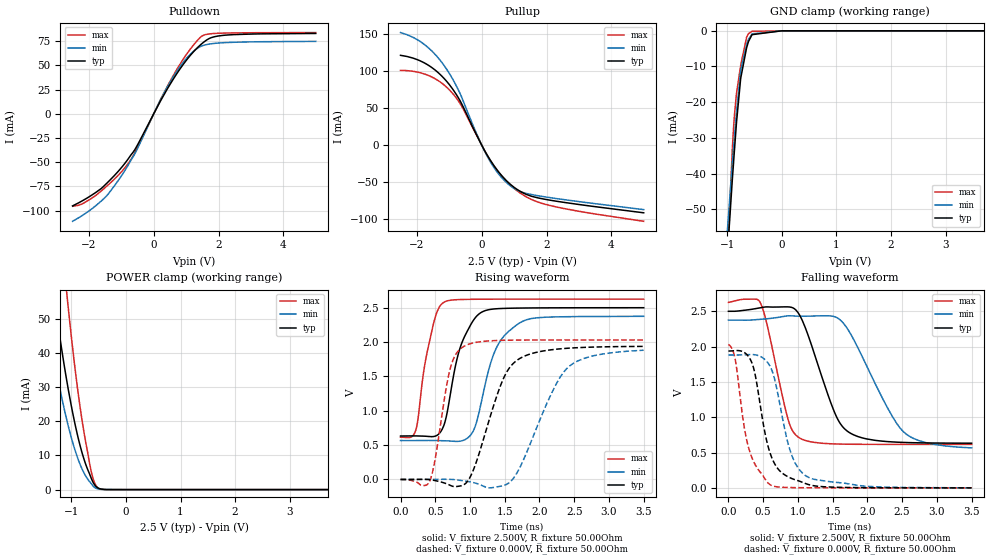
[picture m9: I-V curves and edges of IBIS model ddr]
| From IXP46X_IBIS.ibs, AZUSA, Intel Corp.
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| Note : Termination resitors may be required on pins that are lightly loaded.
|  Correlated with SPICE simulations with Standard JEDEC Test Load
|   |Vref= vcc/2 = 1.250v
|   >
|   < Rref=50ohm
|   >
|   |- Vout
|   _  Cref=30p
[Model]   ddr
Model_type   I/O
Vinl = 940.000mV
Vinh = 1.560V
Vmeas = 1.250V
Rref = 50ohm
Cref = 30.000pF
Vref = 1.250V
|   typ   min   max
C_comp   3.000pF   2.700pF   3.300pF
[Voltage Range]   2.500V   2.375V   2.625V
[Temperature Range]   25.0   110.0   -40.0
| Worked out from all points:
|   slope of the pulldown table from 0 to 0.375 V, typ, clamps not added: 16.3 ohm
|   slope of the pullup table from 0 to 0.375 V, typ, clamps not added: 13.5 ohm
|   POWER clamp passes 1 mA (typ) near -0.55 V on its own axis
|   falling waveform, V_fixture 2.500V, R_fixture 50.00Ohm: 20-80 % time 397ps typ, 564ps min, 269ps max; typ from 2.5 V to 0.632 V
|   rising waveform, V_fixture 2.500V, R_fixture 50.00Ohm: 20-80 % time 268ps typ, 316ps min, 196ps max; typ from 0.632 V to 2.5 V
|   rising waveform, V_fixture 0.000V, R_fixture 50.00Ohm: 20-80 % time 387ps typ, 500ps min, 202ps max; typ from 0 V to 1.94 V
|   falling waveform, V_fixture 0.000V, R_fixture 50.00Ohm: 20-80 % time 247ps typ, 275ps min, 219ps max; typ from 1.94 V to 0 V
[Pulldown]
|   Voltage   I(typ)   I(min)   I(max)
-2.5V     -95.15mA   -111.1mA   -95.57mA
-2.14V    -88.73mA   -103.7mA   -91.89mA
-1.46V    -72.2mA    -85.14mA   -75.16mA
-830mV    -48.59mA   -55.41mA   -53.28mA
-540mV    -34.65mA   -38.67mA   -37.31mA
205mV     12.95mA    14.13mA    14.22mA
475mV     28.81mA    30.99mA    31.72mA
915mV     51.24mA    53.39mA    56.66mA
1.3V      66.68mA    66.53mA    73.99mA
1.525V    73.57mA    70.58mA    80.96mA
1.985V    80.35mA    73.07mA    83.16mA
4.995V    82.99mA    74.82mA    83.91mA
[GND Clamp]
|   Voltage   I(typ)   I(min)   I(max)
-2.5V     -1.132A    -1.076A    -1.37A
-1.035V   -71.78mA   -63.99mA   -77.28mA
-905mV    -41.45mA   -36.81mA   -32.9mA
-885mV    -37.27mA   -33.03mA   -27.5mA
-870mV    -34.01mA   -30.32mA   -24.15mA
-830mV    -25.76mA   -22.9mA    -17.6mA
-750mV    -13.1mA    -10.79mA   -9.436mA
-645mV    -4.789mA   -3.899mA   -1.859mA
-610mV    -3.011mA   -2.375mA   -790.8uA
-545mV    -1.076mA   -850.7uA   -144.4uA
0V        -44.76nA   -10.81nA   -189.7pA
4.995V    0A         0A         0A
[Pullup]
|   Voltage   I(typ)   I(min)   I(max)
-2.5V     121.6mA    152.4mA    101.2mA
-1.71V    109.9mA    134.4mA    95.46mA
-1.315V   97.12mA    116.9mA    86.57mA
-965mV    80.1mA     94.83mA    73.36mA
-625mV    56.68mA    65.86mA    53.33mA
-130mV    11.36mA    12.76mA    11.1mA
205mV     -16.28mA   -17.91mA   -16.18mA
565mV     -38.84mA   -41.59mA   -39.02mA
915mV     -54.43mA   -56.41mA   -55.52mA
1.38V     -67.08mA   -65.74mA   -70.43mA
1.98V     -73.88mA   -70.57mA   -80.68mA
4.995V    -91.99mA   -87.67mA   -103.5mA
[POWER Clamp]
|   Voltage   I(typ)   I(min)   I(max)
-2.5V     245.5mA    188mA      390.5mA
-1.51V    81.13mA    56.98mA    138.7mA
-1.315V   56.33mA    38.27mA    98.46mA
-1.195V   42.88mA    28.35mA    76.14mA
-1.09V    32.38mA    20.76mA    58.4mA
-1.065V   30.07mA    19.12mA    54.44mA
-950mV    20.43mA    12.4mA     37.7mA
-800mV    10.55mA    5.892mA    19.84mA
-635mV    3.283mA    1.746mA    5.211mA
-545mV    862.9uA    386.4uA    1.056mA
-355mV    20.98uA    8.667uA    5.79uA
4.995V    0A         0A         0A
[Ramp]
R_load = 50.00Ohm
|   typ   min   max
dV/dt_r   1.162V/386.825ps   1.129V/498.987ps   1.218V/201.230ps
dV/dt_f   1.121V/397.130ps   1.085V/563.433ps   1.206V/268.614ps
[Falling Waveform]
V_fixture = 2.500V
V_fixture_min = 2.375V
V_fixture_max = 2.625V
R_fixture = 50.00Ohm
|   Time   V(typ)   V(min)   V(max)
0s        2.5V       2.375V     2.625V
460ps     2.55V      2.386V     2.618V
560ps     2.562V     2.395V     2.294V
860ps     2.562V     2.436V     963.4mV
1.03ns    2.436V     2.43V      703.2mV
1.53ns    1.063V     2.423V     622.1mV
1.71ns    803.9mV    2.257V     618.2mV
2.52ns    643.3mV    794.4mV    615.3mV
2.86ns    635.9mV    635.8mV    615.3mV
3.5ns     632.3mV    566mV      615.3mV
[Rising Waveform]
V_fixture = 2.500V
V_fixture_min = 2.375V
V_fixture_max = 2.625V
R_fixture = 50.00Ohm
|   Time   V(typ)   V(min)   V(max)
0s        632.3mV    566mV      615.3mV
220ps     633.6mV    566mV      717.8mV
400ps     626.1mV    568mV      1.931V
630ps     804.7mV    563.2mV    2.582V
870ps     1.953V     559.4mV    2.619V
1.05ns    2.318V     711mV      2.623V
1.17ns    2.436V     1.159V     2.624V
1.39ns    2.485V     1.936V     2.625V
1.75ns    2.495V     2.299V     2.625V
3.5ns     2.5V       2.375V     2.625V
[Rising Waveform]
V_fixture = 0.000V
V_fixture_min = 0.000V
V_fixture_max = 0.000V
R_fixture = 50.00Ohm
|   Time   V(typ)   V(min)   V(max)
0s        529.6nV    121.3nV    3.474nV
420ps     -2.715mV   735.7uV    -23.37mV
500ps     -16.98mV   1.161mV    303.1mV
710ps     -83.03mV   1.5mV      1.592V
910ps     -78.39mV   -20.6mV    1.936V
1.08ns    222.2mV    -53.58mV   1.994V
1.48ns    1.466V     -88.8mV    2.025V
1.66ns    1.722V     67.97mV    2.028V
2.4ns     1.91V      1.621V     2.03V
3.5ns     1.937V     1.881V     2.031V
[Falling Waveform]
V_fixture = 0.000V
V_fixture_min = 0.000V
V_fixture_max = 0.000V
R_fixture = 50.00Ohm
|   Time   V(typ)   V(min)   V(max)
0s        1.937V     1.881V     2.031V
90ps      1.942V     1.881V     1.853V
230ps     1.916V     1.884V     845.7mV
340ps     1.764V     1.887V     422.1mV
600ps     491.3mV    1.72V      45.08mV
720ps     261.1mV    1.286V     12.26mV
900ps     136.8mV    492.7mV    4.468mV
1.14ns    50.49mV    155.2mV    1.509mV
2.01ns    2.128mV    21.13mV    21.96uV
3.5ns     529.6nV    121.3nV    3.474nV
